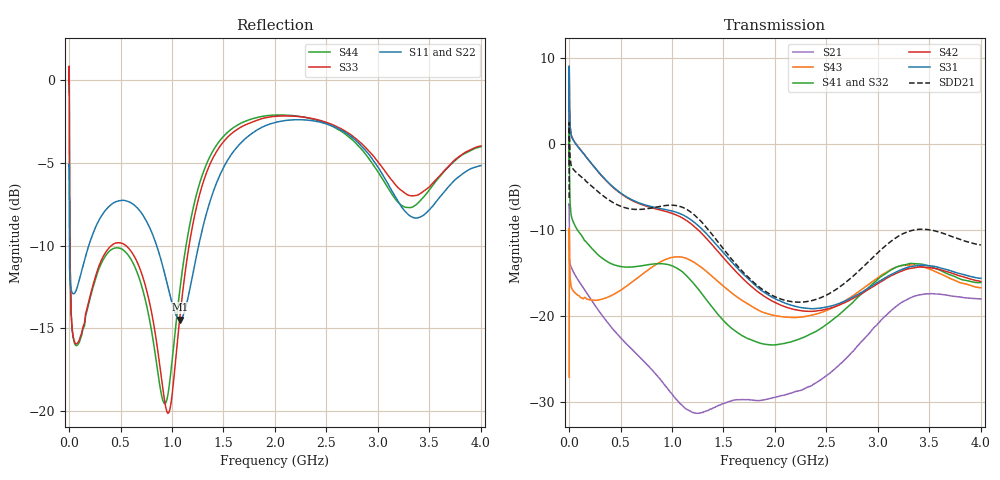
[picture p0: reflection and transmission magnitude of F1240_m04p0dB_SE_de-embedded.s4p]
! Integrated Device Technology
! Corporate Headquarters
! 6024 Silver Creek Valley Road
! San Jose, CA 95138  USA
! Phone:  1-408-284-8200
! Toll Free:  1-800-223-1366
! Webpage:  http://www.idt.com/
! Timing and RF Division
! 515 Groton Road, Suite 102
! Westford, MA 01886-6024
! Device:  F1240
! Description: Dual Intermediate Frequency Digital Variable Gain Amplifier
! Frequency:  10.0 -  500.00 MHz
! Package:  5x5 mm QFN Plastic Package: 32 pin
! Ports:  8 RF, 20 DC
!  Pin  1  = GA3 / Data  Pin 17  = RF OUT_B+
!  Pin  2  = GA4 / CLK  Pin 18  = RF OUT_B-
!  Pin  3  = GA5  Pin 19  = STBY_B
!  Pin  4  = VMODE  Pin 20  = Ground
!  Pin  5  = No Connect  Pin 21  = Ground
!  Pin  6  = GB5  Pin 22  = STB_A
!  Pin  7  = GB4  Pin 23  = RF OUT_A-  = Port 4
!  Pin  8  = GB3  Pin 24  = RF OUT_A+  = Port 3
!  Pin  9  = GB2  Pin 25  = GA0
!  Pin 10  = GB1  Pin 26  = ISET_A
!  Pin 11  = RF IN_B+  Pin 27  = VCC
!  Pin 12  = RF IN_B-  Pin 28  = Ground
!  Pin 13  = Ground  Pin 29  = RF IN_A-  = Port 2
!  Pin 14  = VCC  Pin 30  = RF IN_A+  = Port 1
!  Pin 15  = ISET_B  Pin 31  = GA1
!  Pin 16  = GB0  Pin 32  = GA2 / CSb
! Gain  = +19.5 dB
! State  = 1
! Voltage  = +5.00 V
! Current  = 85.292 mA (one channel only)
! Temperture  =  +25 C
! Test Date  =  2017-10-18
! Board  =  EB4031
! Data:  The device was measured on a custom evaluation board which has
!  individual transmission lines to the RF pins.  Data was collected
!  using a calibrated network analyzer.  The evaluation board was
!  de-embedded using Automatic Fixture Removal.
!  The reference plane is the edge of the package pin.
!  Only Channel A was measured.
!  This data is in single-ended operation.  If your needs are balanced
!  or differential S-parameters then this file needs to be used a
!  linear simulator.
! File Date:  2017-11-10  MJV
! Note:
!  Integrated Device Technology supplies this data as a sample of measured
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# Hz S dB R 100
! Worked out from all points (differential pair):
!   410 points, 500 kHz to 4 GHz, reference 100 ohm
!   strongest paths, dB at 500 kHz, 930 MHz, 1.96 GHz, 2.98 GHz, 4 GHz:
!     S31: 1.8, -7.6, -17.7, -16.2, -15.6
!     S42: 1.8, -7.8, -18.2, -16.4, -16.0
!     S41: -2.5, -13.9, -23.4, -16.0, -16.1
!     S32: -2.5, -14.2, -23.3, -16.3, -16.6
!     S43: -27.1, -13.5, -19.9, -15.7, -16.7
!     S21: -7.0, -28.1, -29.6, -21.2, -18.0
!   taken as a pair (ports 1,2 in; 3,4 out), SDD21 dB: -6.3, -7.2, -17.5, -12.9, -11.7
!   lowest |S11| = -14.5 dB at 1.08 GHz (marker M1), VSWR 1.47, Z = 69.7 - j10.8 ohm
!   |S11| at or under -10 dB: 3.266 MHz to 190.8 MHz (187.5 MHz wide, 193 % of centre); 850.9 MHz to 1.258 GHz (407.6 MHz wide, 38.6 % of centre)
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500000  -5.21 -5.5  -7.03 -5.9  -30.85 79.3  -35.47 77.5
        -7.04 -5.9  -5.20 -5.5  -35.43 76.5  -30.85 80.5
        1.82 -109.1  -2.51 -111.3  -0.21 0.4  -27.13 -39.7
        -2.54 -110.2  1.82 -108.0  -27.13 -39.8  -0.22 2.7
2000000  -7.47 -32.2  -9.84 -33.6  -21.94 26.0  -27.31 6.2
         -9.84 -33.6  -7.45 -32.3  -27.25 5.9  -21.93 26.2
         8.64 -179.2  3.67 163.2  -0.22 -50.9  -9.77 -140.2
         3.62 163.5  8.64 -178.9  -9.77 -140.2  -0.27 -50.6
4000000  -10.76 -28.5  -13.10 -23.5  -22.39 7.6  -30.53 -14.5
         -13.10 -23.6  -10.76 -28.8  -30.49 -14.7  -22.39 7.7
         5.35 158.8  -2.15 138.9  -4.72 -83.4  -12.18 176.4
         -2.20 139.1  5.35 159.0  -12.17 176.3  -4.77 -83.4
3.9e8  -7.62 -139.0  -21.00 -103.0  -26.37 -82.5  -36.23 -63.1
       -21.02 -102.8  -7.51 -140.3  -36.34 -61.7  -26.52 -82.8
       -4.56 57.8  -13.87 11.4  -10.12 -161.3  -17.81 44.7
       -13.81 10.8  -4.61 56.5  -17.74 44.5  -10.34 -161.9
1.08e9  -14.46 -156.7  -30.59 161.7  -25.29 142.6  -32.59 -176.6
        -30.25 160.7  -14.49 -154.6  -32.56 -172.1  -26.14 142.2
        -8.09 -102.7  -14.90 165.9  -14.10 -106.2  -13.30 -140.5
        -14.69 161.3  -8.46 -105.2  -13.13 -140.4  -12.47 -106.1
2.86e9  -4.11 101.9  -22.81 -26.4  -26.41 -152.7  -28.65 -137.1
        -22.75 -26.4  -3.86 102.7  -29.40 -124.5  -27.68 -146.9
        -17.11 -65.5  -17.61 -149.5  -3.94 102.0  -17.60 -82.4
        -17.25 -160.2  -17.28 -62.4  -16.77 -79.9  -4.31 95.1
4e9  -5.15 -134.8  -18.03 110.3  -25.07 -38.6  -26.10 -23.0
     -18.02 110.2  -4.82 -133.4  -26.88 -7.9  -26.87 -31.2
     -15.63 44.2  -16.61 -57.6  -3.97 -133.7  -18.26 64.7
     -16.12 -71.3  -15.99 50.0  -16.72 56.9  -4.02 -143.5
